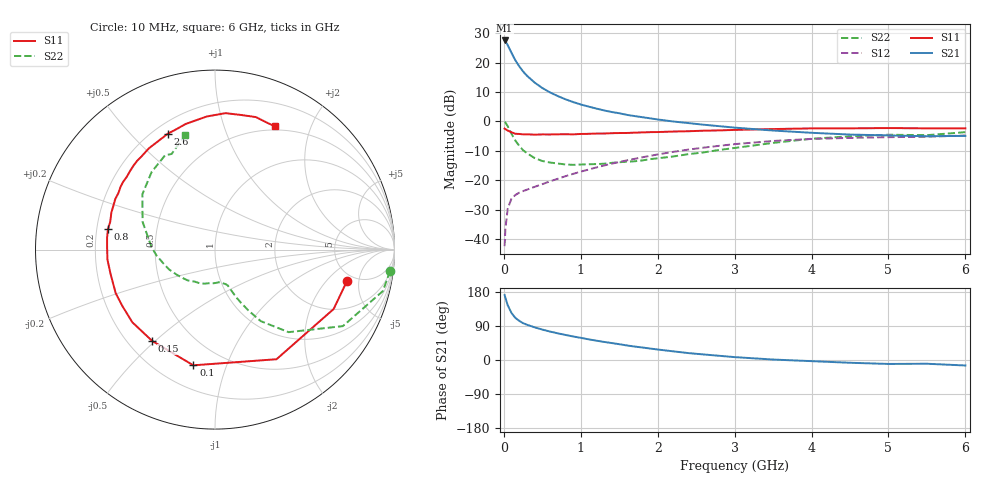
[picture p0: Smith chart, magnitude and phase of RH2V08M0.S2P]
! SIEMENS Small Signal Semiconductors
! BFR106
! Si NPN RF Bipolar Junction Transistor in SOT23
! VCE = 2 V  IC = 8 mA
! Common Emitter S-Parameters:  August  1996
# GHz  S  MA  R  50
!  f  S11  S21  S12  S22
! GHz  MAG  ANG  MAG  ANG  MAG  ANG  MAG  ANG
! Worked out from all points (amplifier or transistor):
!   36 points, 10 MHz to 6 GHz, reference 50 ohm
!   highest |S21| = 27.5 dB at 10 MHz (marker M1)
!   |S21| within 3 dB of that: start of sweep to 76.93 MHz
!   unconditionally stable (mu >= 1): 512.5 MHz to 2.304 GHz; 4.428 GHz to end of sweep
!   at 250 MHz: K = 0.65, MSG = 20.3 dB, |S12| = -23.7 dB
!   at 1.4 GHz: K = 1.12, MAG = 6.7 dB, |S12| = -14.4 dB
!   at 6 GHz: K = 1.02, MAG = -0.9 dB, |S12| = -4.8 dB
!   S11 on the Smith chart (normalised r, x): 10 MHz: 4.20, -3.47; 100 MHz: 0.34, -0.77; 150 MHz: 0.30, -0.49; 800 MHz: 0.25, +0.09; 2.6 GHz: 0.26, +0.64; 6 GHz: 0.46, +1.50
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0.01  0.7553 -13.6  23.8 171.4  0.0076 84.7  0.9827 -7.0
0.02  0.7393 -26.6  23.18 164.5  0.0148 76.4  0.9632 -13.9
0.05  0.7004 -60.7  19.89 144.6  0.0328 62.2  0.8303 -30.9
0.1  0.6559 -100.6  14.62 123.9  0.0493 48.1  0.6161 -48.3
0.15  0.6176 -124.6  10.93 111.0  0.0564 42.4  0.4729 -57.4
0.2  0.6133 -138.7  8.669 103.3  0.0616 41.2  0.3856 -61.3
0.25  0.6043 -149.0  7.072 97.2  0.0655 40.9  0.3247 -64.2
0.3  0.6041 -156.4  5.991 93.1  0.0693 42.6  0.2888 -66.1
0.4  0.5975 -167.2  4.588 86.2  0.0774 45.4  0.2389 -68.6
0.5  0.6019 -174.8  3.7 80.3  0.086 48.3  0.2128 -70.3
0.6  0.6011 179.0  3.118 75.1  0.096 50.8  0.2007 -73.0
0.8  0.6073 169.1  2.385 66.2  0.1173 54.4  0.1862 -80.2
0.9  0.6038 165.2  2.138 62.1  0.1287 55.8  0.183 -83.5
1.1  0.6164 156.7  1.791 54.6  0.1523 57.1  0.1876 -92.5
1.3  0.6235 149.7  1.543 47.8  0.1782 57.2  0.1913 -101.5
1.6  0.6375 140.3  1.294 38.4  0.2184 56.0  0.2071 -116.5
2.2  0.674 123.1  1 22.9  0.3041 49.9  0.2538 -146.1
2.6  0.6972 112.2  0.88 14.6  0.3594 44.0  0.2986 -165.3
3.5  0.7429 93.6  0.701 1.2  0.4664 28.9  0.4323 159.0
4.5  0.7642 78.8  0.599 -7.3  0.5258 12.0  0.5584 129.2
5.5  0.764 67.6  0.561 -9.9  0.5508 1.7  0.5852 114.4
6  0.7636 64.1  0.569 -14.5  0.5763 -5.6  0.6579 104.8
